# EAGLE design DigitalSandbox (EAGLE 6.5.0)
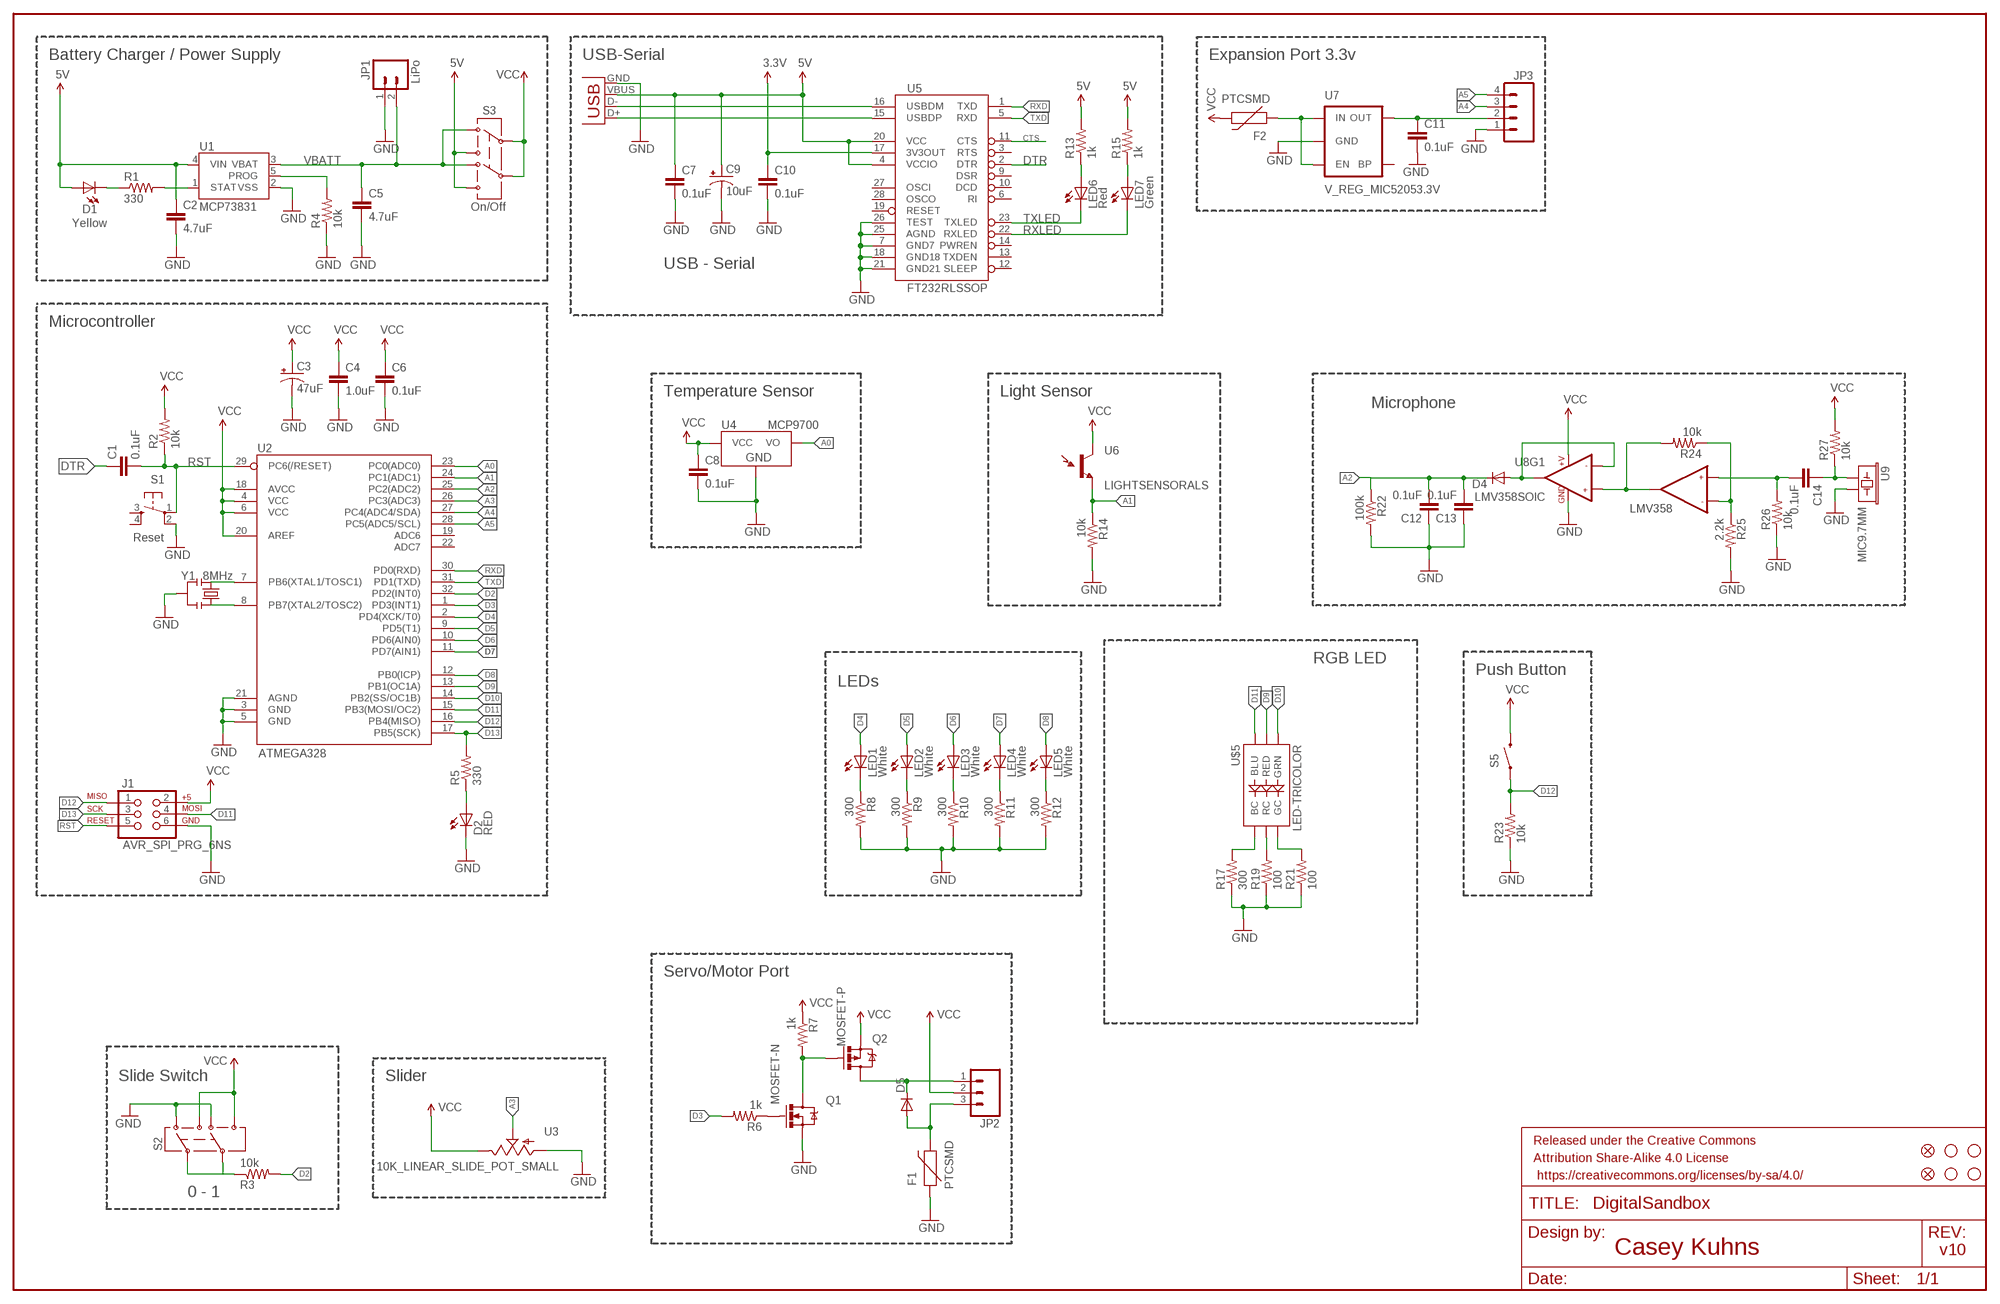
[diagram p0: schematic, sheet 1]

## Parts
C1  0.1uF  0.1UF-25V(+80/-20%)(0603)  [0603-CAP]
C2  4.7uF  4.7UF-6.3V-10%(0603)0603  [0603-CAP]
C3  47uF  47UF-10V-10%(TANT)  [EIA3528]
C4  1.0uF  1.0UF-16V-10%(0603)  [0603-CAP]
C5  4.7uF  4.7UF-6.3V-10%(0603)0603  [0603-CAP]
C6  0.1uF  0.1UF-25V(+80/-20%)(0603)  [0603-CAP]
C7  0.1uF  0.1UF-25V(+80/-20%)(0603)  [0603-CAP]
C8  0.1uF  0.1UF-25V(+80/-20%)(0603)  [0603-CAP]
C9  10uF  10UF-16V-10%(TANT)  [EIA3216]
C10  0.1uF  0.1UF-25V(+80/-20%)(0603)  [0603-CAP]
C11  0.1uF  0.1UF-25V(+80/-20%)(0603)  [0603-CAP]
C12  0.1uF  0.1UF-25V(+80/-20%)(0603)  [0603-CAP]
C13  0.1uF  0.1UF-25V(+80/-20%)(0603)  [0603-CAP]
C14  0.1uF  0.1UF-25V(+80/-20%)(0603)  [0603-CAP]
D1  Yellow  LED-YELLOW0603  [LED-0603]
D2  RED  LED-RED1206  [LED-1206]
D4  DIODESOD  [SOD-323]
D5  DIODESOD  [SOD-323]
F1  PTCSMD  [PTC-1206]
F2  PTCSMD  [PTC-1206]
FID1  FIDUCIAL1X2  [FIDUCIAL-1X2]
FID2  FIDUCIAL1X2  [FIDUCIAL-1X2]
FRAME1  FRAME-LEDGER  [CREATIVE_COMMONS]
J1  AVR_SPI_PRG_6NS  [2X3-NS]
JP1  LiPo  M02-JST-2MM-SMT  [JST-2-SMD]
JP2  M03SMD_RA_FEMALE  [1X03_SMD_RA_FEMALE]
JP3  M04SMD_STRAIGHT_COMBO  [1X04_SMD_STRAIGHT_COMBO]
LED1  White  LED-WHITE  [LED-1206]
LED2  White  LED-WHITE  [LED-1206]
LED3  White  LED-WHITE  [LED-1206]
LED4  White  LED-WHITE  [LED-1206]
LED5  White  LED-WHITE  [LED-1206]
LED6  Red  LED-RED0603  [LED-0603]
LED7  Green  LED-GREEN0603  [LED-0603]
Q1  MOSFET-N  MOSFET-NCHANNELBSS138  [SOT23]
Q2  MOSFET-P  MOSFET-PCHANNEL  [SOT23-3]
R1  330  330OHM1/10W1%(0603)  [0603-RES]
R2  10k  10KOHM1/10W1%(0603)0603  [0603-RES]
R3  10k  10KOHM1/10W1%(0603)0603  [0603-RES]
R4  10k  10KOHM1/10W1%(0603)0603  [0603-RES]
R5  330  330OHM1/10W1%(0603)  [0603-RES]
R6  1k  1KOHM1/10W1%(0603)  [0603-RES]
R7  1k  1KOHM1/10W1%(0603)  [0603-RES]
R8  300  300OHM-1/10W-1%(0603)  [0603-RES]
R9  300  300OHM-1/10W-1%(0603)  [0603-RES]
R10  300  300OHM-1/10W-1%(0603)  [0603-RES]
R11  300  300OHM-1/10W-1%(0603)  [0603-RES]
R12  300  300OHM-1/10W-1%(0603)  [0603-RES]
R13  1k  1KOHM1/10W1%(0603)  [0603-RES]
R14  10k  10KOHM1/10W1%(0603)0603  [0603-RES]
R15  1k  1KOHM1/10W1%(0603)  [0603-RES]
R17  300  300OHM-1/10W-1%(0603)  [0603-RES]
R19  100  100OHM1/10W1%(0603)  [0603-RES]
R21  100  100OHM1/10W1%(0603)  [0603-RES]
R22  100k  100KOHM1/10W1%(0603)  [0603-RES]
R23  10k  10KOHM1/10W1%(0603)0603  [0603-RES]
R24  10k  10KOHM1/10W1%(0603)0603  [0603-RES]
R25  2.2k  2.2KOHM1/10W1%(0603)  [0603-RES]
R26  10k  10KOHM1/10W1%(0603)0603  [0603-RES]
R27  10k  10KOHM1/10W1%(0603)0603  [0603-RES]
S1  Reset  TAC_SWITCHSMD  [TACTILE_SWITCH_SMD]
S2  SWITCH-DPDTAYZ0202  [AYZ0202]
S3  On/Off  SWITCH-DPDTAYZ0202  [AYZ0202]
S5  SWITCH-MOMENTARY-2SMD-4  [TACTILE_SWITCH_TALL]
STANDOFF1  STAND-OFF  [STAND-OFF]
STANDOFF2  STAND-OFF  [STAND-OFF]
STANDOFF3  STAND-OFF  [STAND-OFF]
STANDOFF4  STAND-OFF  [STAND-OFF]
U1  MCP73831  [SOT23-5]
U2  ATMEGA328  ATMEGA328_SMT  [TQFP32-08]
U3  10K_LINEAR_SLIDE_POT_SMALL  [C2031N-1A2-B10K-GP]
U4  MCP9700  MCP9700SMD  [SOT23-3]
U5  FT232RLSSOP  [SSOP28DB]
U6  LIGHTSENSORALS  [ALS-PT19]
U7  V_REG_MIC52053.3V  [SOT23-5]
U8  LMV358SOIC  [SO08]
U9  MIC9.7MM  [MIC-9.7MM]
U$5  LED-TRICOLOR  LED-TRICOLOR-NO-COMPLCC-6-SMD  [PLCC-6-LED]
X1  USBSMD  [USB-MINIB]
Y1  8MHz  RESONATOR8MHZ  [RESONATOR-SMD]

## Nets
3.3V [power]: C10.1 U5.17(3V3OUT)
5V: C2.1 C7.1 C9.A(+) D1.A R13.2 R15.2 S3.3 S3.6 U1.4(VIN) U5.4(VCCIO) U5.20(VCC) X1.VBUS
A0: U2.23(PC0(ADC0)) U4.2(VO)
A1: R14.1 U2.24(PC1(ADC1)) U6.E(E1)
A2: C12.2 C13.2 D4.C R22.1 U2.25(PC2(ADC2))
A3: U2.26(PC3(ADC3)) U3.1(S)
A4: JP3.3 U2.27(PC4(ADC4/SDA))
A5: JP3.4 U2.28(PC5(ADC5/SCL))
BLUE: R17.2 U$5.CB(BC)
CTS: U5.11(CTS)
D2: R3.2 U2.32(PD2(INT0))
D3: R6.2 U2.1(PD3(INT1))
D4: LED1.A U2.2(PD4(XCK/T0))
D5: LED2.A U2.9(PD5(T1))
D6: LED3.A U2.10(PD6(AIN0))
D7: LED4.A U2.11(PD7(AIN1))
D8: LED5.A U2.12(PB0(ICP))
D9: U2.13(PB1(OC1A)) U$5.AR(RED)
D10: U2.14(PB2(SS/OC1B)) U$5.AG(GRN)
D11: J1.4 U2.15(PB3(MOSI/OC2)) U$5.AB(BLU)
D12: J1.1 R23.2 S5.A2 U2.16(PB4(MISO))
D13: J1.3 R5.2 U2.17(PB5(SCK))
DTR: C1.1 U5.2(DTR)
GND [power]: C2.2 C3.C(-) C4.2 C5.2 C6.2 C7.2 C8.2 C9.C(-) C10.2 C11.2 C12.1 C13.1 D2.C F1.1 J1.6 JP1.1 JP3.1 Q1.2(S) R4.1 R8.2 R9.2 R10.2 R11.2 R12.2 R14.2 R17.1 R19.1 R21.1 R22.2 R23.1 R25.2 R26.1 S1.2 S2.1 S2.4 U1.2(VSS) U2.3(GND) U2.5(GND) U2.21(AGND) U3.2(A) U4.3(GND) U5.7(GND7) U5.18(GND18) U5.21(GND21) U5.25(AGND) U5.26(TEST) U7.2(GND) U8.4(GND) U9.2 X1.GND Y1.2
GRN: R21.2 U$5.CG(GC)
N$1: U2.7(PB6(XTAL1/TOSC1)) Y1.1
N$2: D2.A R5.1
N$3: U2.8(PB7(XTAL2/TOSC2)) Y1.3
N$4: Q1.3(D) Q2.1(G) R7.2
N$5: LED6.A R13.1
N$6: LED7.A R15.1
N$7 [power]: F2.1 U7.1(IN) U7.3(EN)
N$8: D5.C JP2.1 Q2.3(D)
N$9: LED3.C R10.1
N$10: Q1.1(G) R6.1
N$11: LED4.C R11.1
N$12: C11.1 JP3.2 U7.5(OUT)
N$13: LED5.C R12.1
N$15: R3.1 S2.2 S2.5
N$16 [power]: D5.A F1.2 JP2.3
N$17: C14.1 R27.1 U9.1
N$18: LED1.C R8.1
N$20: C14.2 R26.2 U8.5(+IN2)
N$21: LED2.C R9.1
N$23: R24.1 R25.1 U8.6(-IN2)
N$24: D4.A U8.1(OUT1) U8.2(-IN1)
N$26: R24.2 U8.3(+IN1) U8.7(OUT2)
N$33: D1.C R1.1
PROG: R4.2 U1.5(PROG)
RED: R19.2 U$5.CR(RC)
RST: C1.2 J1.5 R2.1 S1.1 U2.29(PC6(/RESET))
RXD: U2.30(PD0(RXD)) U5.1(TXD)
RXLED: LED7.C U5.22(RXLED)
STAT: R1.2 U1.1(STAT)
TXD: U2.31(PD1(TXD)) U5.5(RXD)
TXLED: LED6.C U5.23(TXLED)
USB_D+: U5.15(USBDP) X1.D+
USB_D-: U5.16(USBDM) X1.D-
VBATT: C5.1 JP1.2 S3.1 S3.4 U1.3(VBAT)
VCC [power]: C3.A(+) C4.1 C6.1 C8.1 F2.2 J1.2 JP2.2 Q2.2(S) R2.2 R7.1 R27.2 S2.3 S2.6 S3.2 S3.5 S5.B2 U2.4(VCC) U2.6(VCC) U2.18(AVCC) U2.20(AREF) U3.3(E) U4.1(VCC) U6.C(C1) U8.8(+V)
Unconnected: S1.3 S1.4 U2.19(ADC6) U2.22(ADC7) U5.3(RTS) U5.6(RI) U5.9(DSR) U5.10(DCD) U5.12(SLEEP) U5.13(TXDEN) U5.14(PWREN) U5.19(RESET) U5.27(OSCI) U5.28(OSCO) U7.4(BP)

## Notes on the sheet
- Battery Charger / Power Supply | USB-Serial | Expansion Port 3.3v
- USB - Serial
- Microcontroller
- Temperature Sensor | Light Sensor
- Microphone
- LMV358
- RGB LED
- Push Button
- LEDs
- Servo/Motor Port
- Slide Switch | Slider
- 0 - 1
- Casey Kuhns | v10

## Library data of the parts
C1 C6-C8 C10-C14 = SparkFun-Capacitors:0.1UF-25V(+80/-20%)(0603): CAP-00810; PROD_ID: CAP-00810
C2 C5 = SparkFun-Capacitors:4.7UF-6.3V-10%(0603): CAP-08280; PROD_ID: CAP-08280
C3 = SparkFun-Capacitors:47UF-10V-10%(TANT): CAP-08310; PROD_ID: CAP-08310
C4 = SparkFun-Capacitors:1.0UF-16V-10%(0603): CAP-00868; PROD_ID: CAP-00868
C9 = SparkFun-Capacitors:10UF-16V-10%(TANT): CAP-00811; PROD_ID: CAP-00811
D1 = SparkFun-LED:LED-YELLOW: Yellow SMD LEDs; PROD_ID: DIO-09003
D2 = SparkFun-LED:LED-RED: Assorted Red LEDs; PROD_ID: DIO-00809
D4 D5 = SparkFun-DiscreteSemi:DIODE: Diode; PROD_ID: DIO-09646
F1 F2 = SparkFun-PowerIC:PTC: Resettable Fuse PTC; PROD_ID: RES-11150
FID1 FID2 = SparkFun-Aesthetics:FIDUCIAL: Fiducial Alignment Points
FRAME1 = SparkFun-Aesthetics:FRAME-LEDGER: Schematic Frame
J1 = SparkFun-Connectors:AVR_SPI_PRG_6: AVR ISP 6 Pin This is the reduced ISP connector for AVR programming. Common on Arduino. This footprint will take up less PCB space and can be used with a 10-pin to 6-pin adapter such as SKU: BOB-08508
JP1 = SparkFun-Connectors:M02: Standard 2-pin 0.1" header. Use with; PROD_ID: CONN-08352
JP2 = SparkFun-Connectors:M03: Header 3 Standard 3-pin 0.1" header. Use with straight break away headers (SKU : PRT-00116), right angle break away headers (PRT-00553), swiss pins (PRT-00743), machine pins (PRT-00117), and female headers (PRT-00115). Molex polarized connector foot print use with SKU : PRT-08232 with associated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; PROD_ID: CONN-10926; VALUE: 1x3 RA Female .1"
JP3 = SparkFun-Connectors:M04: Header 4 Standard 4-pin 0.1" header. Use with straight break away headers (SKU : PRT-00116), right angle break away headers (PRT-00553), swiss pins (PRT-00743), machine pins (PRT-00117), and female headers (PRT-00115). Molex polarized connector foot print use with SKU : PRT-08231 with associated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
LED1-LED5 = SparkFun-LED:LED-WHITE: White SMD LEDs; PROD_ID: DIO-09955; VALUE: WHITE
LED6 = SparkFun-LED:LED-RED: Assorted Red LEDs; PROD_ID: DIO-00819; VALUE: RED
LED7 = SparkFun-LED:LED-GREEN: Various green LEDs; PROD_ID: DIO-00821; VALUE: GREEN
Q1 = SparkFun-DiscreteSemi:MOSFET-NCHANNEL: Common NMOSFET Parts MFG P/NStore IDProd ID FDD8780TRANS-09984 SI7820DNTRANS-11055 FDS6630AIC-08089 2N7002PWTRANS-11151 FQP30N06L COM-10213TRANS-10060 BSS123LT1GTRANS-08345 BSS138TRANS-00830 BS170 2N7000; PROD_ID: TRANS-00830
Q2 = SparkFun-DiscreteSemi:MOSFET-PCHANNEL: Generic PMOSFET; PROD_ID: TRANS-08285
R1 R5 = SparkFun-Resistors:330OHM1/10W1%(0603): RES-00818; PROD_ID: RES-00818
R2-R4 R14 R23 R24 R26 R27 = SparkFun-Resistors:10KOHM1/10W1%(0603): RES-00824; PROD_ID: RES-00824; VALUE: 10K
R6 R7 R13 R15 = SparkFun-Resistors:1KOHM1/10W1%(0603): RES-07856; PROD_ID: RES-07856; VALUE: 1K
R8-R12 R17 = SparkFun-Resistors:300OHM-1/10W-1%(0603): RES-10328; PROD_ID: RES_10328
R19 R21 = SparkFun-Resistors:100OHM1/10W1%(0603): RES-07863; PROD_ID: RES-07863
R22 = SparkFun-Resistors:100KOHM1/10W1%(0603): RES-07828; PROD_ID: RES-07828
R25 = SparkFun-Resistors:2.2KOHM1/10W1%(0603): RES-08272; PROD_ID: RES-08272
S1 = SparkFun-Electromechanical:TAC_SWITCH: Momentary Switch Button commonly used for reset or general input. Spark Fun Electronics SKU : COM-00097 SMT- SWCH-08247; PROD_ID: SWCH-08247
S2 S3 = SparkFun-Electromechanical:SWITCH-DPDT: DPDT Version of the COM-00597; PROD_ID: SWCH-08179; VALUE: DPDT
S5 = SparkFun-Electromechanical:SWITCH-MOMENTARY-2: Various NO switches- pushbuttons, reed, etc; PROD_ID: SWCH-11966
STANDOFF1-STANDOFF4 = SparkFun-Electromechanical:STAND-OFF: #4 Stand Off
U1 = SparkFun-PowerIC:MCP73831: Miniature single cell, fully integrated Li-Ion, Li-polymer charge management controller http://ww1.microchip.com/downloads/en/DeviceDoc/21984a.pdf IC-09995; PROD_ID: IC-09995
U2 = SparkFun-DigitalIC:ATMEGA328_SMT: 32-Pin Atmega328 part Commonly used on Arduino compatible boards Available in QFP and QFN packages TQFP is IC-09069 QFN is non-stock; PROD_ID: IC-09069; VALUE: ATMEGA328P
U3 = SparkFun-Resistors:10K_LINEAR_SLIDE_POT_SMALL; PROD_ID: RES-11924
U4 = SparkFun-Sensors:MCP9700: Analog-output temperature sensor; PROD_ID: IC-08917
U5 = SparkFun-DigitalIC:FT232RL: USB UART FT232RL 4th Generation USB UART (USB <-> Serial) Controller. Spark Fun Electronics SKU : COM-00650 Production SKU IC-00870; PROD_ID: IC-00870
U6 = SparkFun-Sensors:LIGHTSENSOR: Ambient Light Sensor; PROD_ID: IC-11836
U7 = SparkFun-PowerIC:V_REG_MIC5205: V_REG MIC5219 Standard 3.3V and 5V 150mA LDO voltage regulator in SOT-23 layout. Micrel part MIC5205. BP (by-pass) pin is used to lower output noise with 470pF cap, may be left open.; PROD_ID: VREG-00822; VALUE: 3.3V/150mA
U8 = SparkFun-AnalogIC:LMV358: Jellybean rail-to-rail output op-amp; PROD_ID: IC-09657
U9 = SparkFun-Sensors:MIC: Omni-directional electret microphone. 9.7mm standard diameter.; PROD_ID: COMP-08856
U$5 = SparkFun-LED:LED-TRICOLOR-NO-COM; PROD_ID: DIO-12113
X1 = SparkFun-Connectors:USB: USB Connectors USB-B-PTH is fully proven SKU : PRT-00139/CONN-08278 USB-miniB is fully proven SKU : PRT-00587 USB-A-PCB is untested. USB-A-H is throughly reviewed, but untested. Spark Fun Electronics SKU : PRT-00437 USB-B-SMT is throughly reviewed, but untested. Needs silkscreen touching up.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; PROD_ID: CONN-08193
Y1 = SparkFun-FreqCtrl:RESONATOR: Resonator Small SMD resonator. Used, eg, on the Arduino Pro/ Pro Mini boards. 8MHz- XTAL-08895 16MHz- XTAL-08900; PROD_ID: XTAL-08895; VALUE: 8MHZ

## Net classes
0 default: width 0.203 mm
1 power: width 0.254 mm

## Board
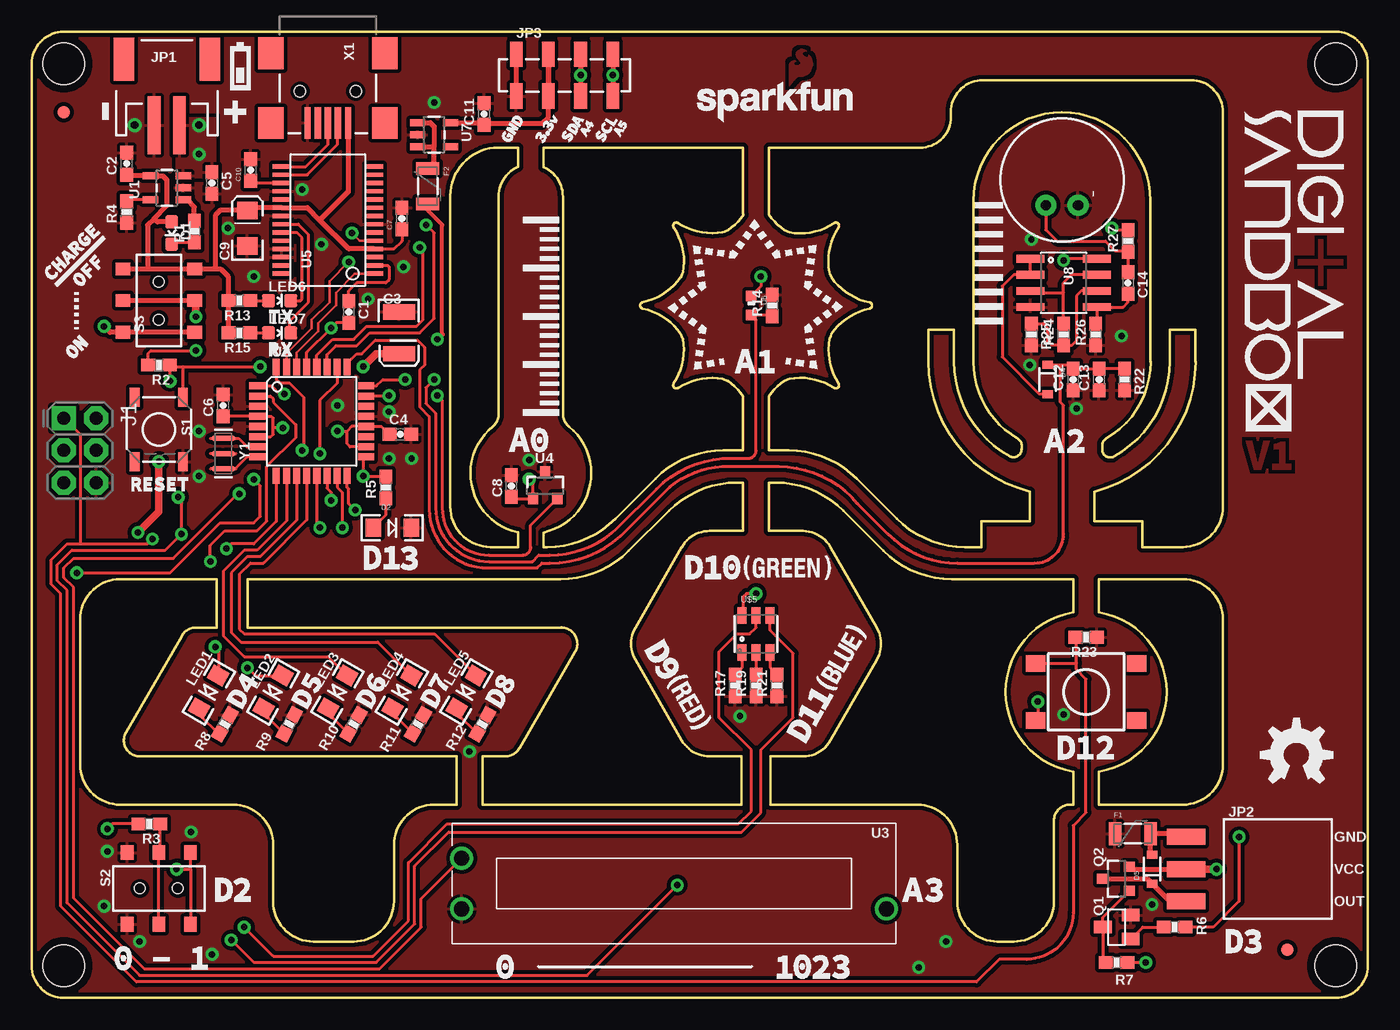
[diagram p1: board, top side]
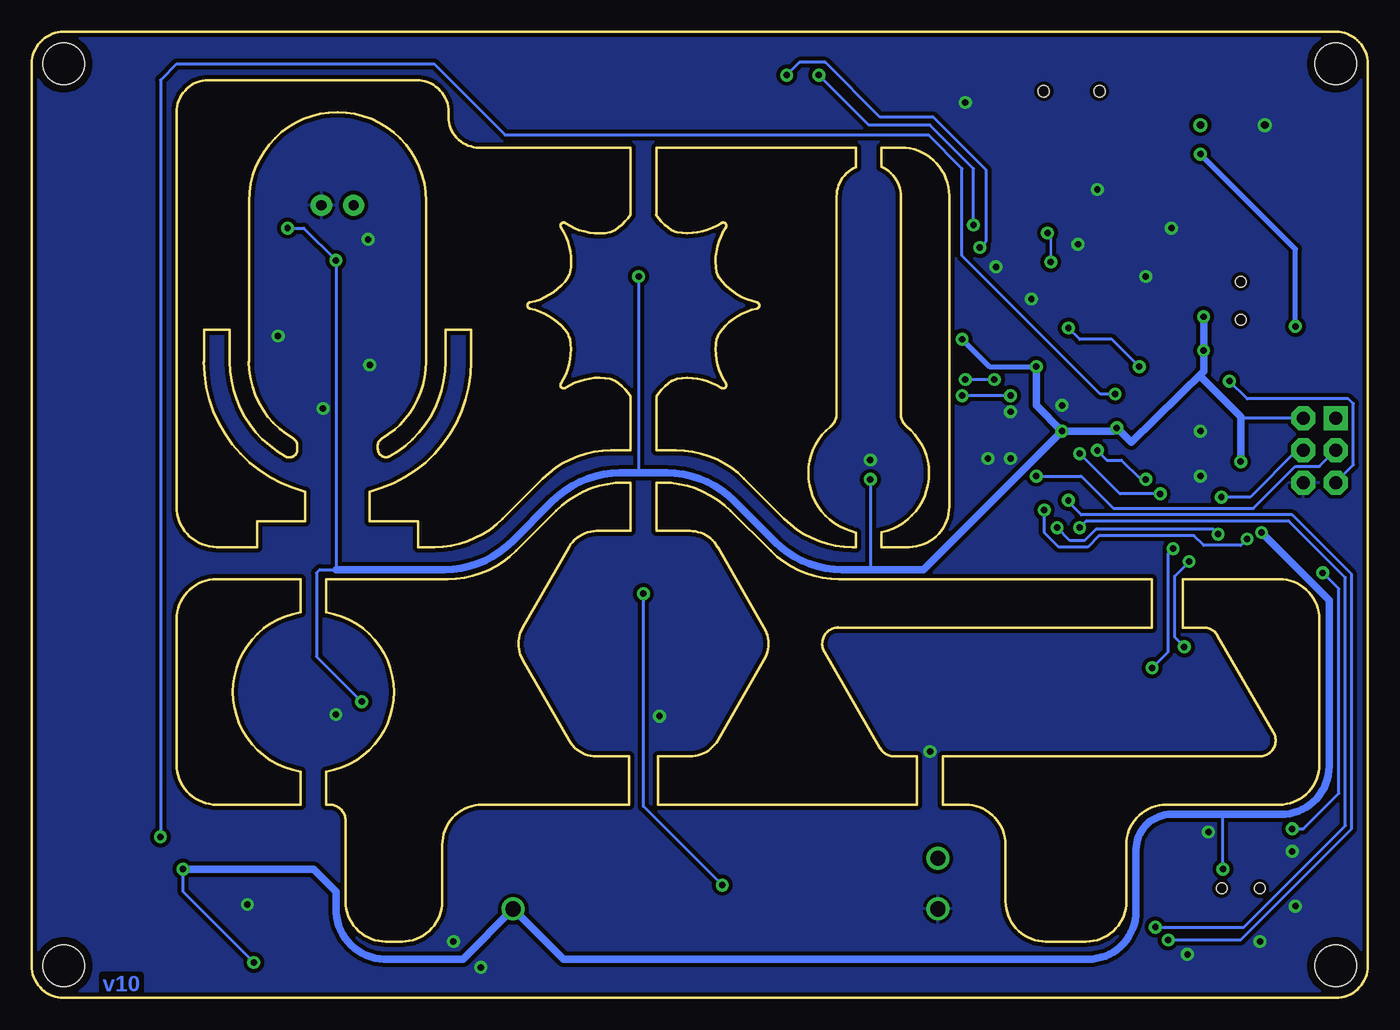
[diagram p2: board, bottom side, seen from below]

Size 105.41 x 76.2 mm. Coordinates in mm from the lower left corner, seen from the top.
Outline: 182 segments
Copper layers (1*16): Top 0.035mm / dielectric 1.5mm / Bottom 0.035mm
Design rules "SparkFun-2-layer": minimum track width 7mil, minimum drill 15mil, track to track 8mil, track to pad 8mil, pad to pad 8mil, via to via 8mil, smd to smd 8mil, copper to edge 8mil, drill to drill 8mil, minimum pad ring 12mil, minimum via ring 10mil, stop-mask expansion 4mil, vias tented up to drill 20mil, thermal gap 10mil

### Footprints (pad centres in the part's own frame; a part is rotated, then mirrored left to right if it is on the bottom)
0603-CAP = smd 1.1 x 1: 1 -0.85,0; 2 0.85,0
EIA3528 = smd 1.2 x 2.5: A 1.65,0; C -1.65,0
EIA3216 = smd 1.4 x 1.6: A 1.4,0; C -1.4,0
LED-0603 = smd 1 x 1: A 0,-0.877; C 0,0.877
LED-1206 = smd 1.2 x 1.4: A -1.5,0; C 1.5,0
SOD-323 = smd 0.63 x 0.83: A 1.15,0; C -1.15,0
PTC-1206 = smd 1 x 1.8: 1 -1.4,0; 2 1.4,0
FIDUCIAL-1X2 = smd 1 x 1: 1 0,0
2X3-NS = drill 1.016 pad 1.88 square: 1 -2.54,-1.27 | drill 1.016 pad 1.88 octagon: 2 -2.54,1.27; 3 0,-1.27; 4 0,1.27; 5 2.54,-1.27; 6 2.54,1.27
JST-2-SMD = smd 1 x 4.6: 1 -1,-3.7; 2 1,-3.7 | smd 1.6 x 3.4: NC1 -3.4,1.5; NC2 3.4,1.5
1X03_SMD_RA_FEMALE = smd 1.25 x 3: 1 -2.54,7.225; 2 0,7.225; 3 2.54,7.225
1X04_SMD_STRAIGHT_COMBO = smd 1 x 2: 1 0,-1.65; 1-2 0,1.65; 2 2.54,1.65; 2-2 2.54,-1.65; 3 5.08,-1.65; 3-2 5.08,1.65; 4 7.62,1.65; 4-2 7.62,-1.65
SOT23 = smd 1 x 1.4: 1 -0.95,-1.1; 2 0.95,-1.1; 3 0,1.1
SOT23-3 = smd 0.8 x 0.9: 1 -0.95,-1; 2 0.95,-1; 3 0,1.1
0603-RES = smd 1.1 x 1: 1 -0.85,0; 2 0.85,0
TACTILE_SWITCH_SMD = smd 1.524 x 0.762: 1 -2.54,1.905; 2 2.54,1.905; 3 -2.54,-1.905; 4 2.54,-1.905
AYZ0202 = smd 1 x 1.15: 1 -2.5,2.825; 2 0,2.825; 3 2.5,2.825; 4 -2.5,-2.825; 5 0,-2.825; 6 2.5,-2.825 | hole 0.85: 1.5,0; -1.5,0
TACTILE_SWITCH_TALL = smd 1.55 x 1.3: A1 -3.975,-2.25; A2 3.975,-2.25; B1 -3.975,2.25; B2 3.975,2.25
STAND-OFF = hole 3.302: 0,0
SOT23-5 = smd 0.55 x 1.2: 1 -0.95,-1.3; 2 0,-1.3; 3 0.95,-1.3; 4 0.95,1.3; 5 -0.95,1.3
TQFP32-08 = smd 1.27 x 0.559: 1 -4.293,2.8; 2 -4.293,2; 3 -4.293,1.2; 4 -4.293,0.4; 5 -4.293,-0.4; 6 -4.293,-1.2; 7 -4.293,-2; 8 -4.293,-2.8; 17 4.293,-2.8; 18 4.293,-2; 19 4.293,-1.2; 20 4.293,-0.4; 21 4.293,0.4; 22 4.293,1.2; 23 4.293,2; 24 4.293,2.8 | smd 0.559 x 1.27: 9 -2.8,-4.293; 10 -2,-4.293; 11 -1.2,-4.293; 12 -0.4,-4.293; 13 0.4,-4.293; 14 1.2,-4.293; 15 2,-4.293; 16 2.8,-4.293; 25 2.8,4.293; 26 2,4.293; 27 1.2,4.293; 28 0.4,4.293; 29 -0.4,4.293; 30 -1.2,4.293; 31 -2,4.293; 32 -2.8,4.293
C2031N-1A2-B10K-GP = drill 1.2: 1 -16.75,2; 2 -16.75,-2; 3 16.75,-2
SSOP28DB = smd 0.348 x 1.397: 1 -4.225,-3.656; 2 -3.575,-3.656; 3 -2.925,-3.656; 4 -2.275,-3.656; 5 -1.625,-3.656; 6 -0.975,-3.656; 7 -0.325,-3.656; 8 0.325,-3.656; 9 0.975,-3.656; 10 1.625,-3.656; 11 2.275,-3.656; 12 2.925,-3.656; 13 3.575,-3.656; 14 4.225,-3.656; 15 4.225,3.656; 16 3.575,3.656; 17 2.925,3.656; 18 2.275,3.656; 19 1.625,3.656; 20 0.975,3.656; 21 0.325,3.656; 22 -0.325,3.656; 23 -0.975,3.656; 24 -1.625,3.656; 25 -2.275,3.656; 26 -2.925,3.656; 27 -3.575,3.656; 28 -4.225,3.656
ALS-PT19 = smd 0.8 x 0.8: C -0.75,0; E 0.75,0
SO08 = smd 0.61 x 2.21: 1 -1.905,-2.616; 2 -0.635,-2.616; 3 0.635,-2.616; 4 1.905,-2.616; 5 1.905,2.616; 6 0.635,2.616; 7 -0.635,2.616; 8 -1.905,2.616
MIC-9.7MM = drill 0.8 pad 1.676: 1 -2,1.27; 2 -2,-1.27
PLCC-6-LED = smd 0.7 x 1.3: AB -1.1,1.475; AG 1.1,1.475; AR 0,1.475; CB -1.1,-1.475; CG 1.1,-1.475; CR 0,-1.475
USB-MINIB = smd 2.5 x 0.5: D+ 2.5,0; D- 2.5,0.8; GND 2.5,-1.6; ID 2.5,-0.8; VBUS 2.5,1.6 | smd 2.5 x 2: MTN1 -3,4.5; MTN2 2.5,4.5; MTN3 -3,-4.5; MTN4 2.5,-4.5 | hole 0.9: 0,2.2; 0,-2.2
RESONATOR-SMD = smd 0.45 x 1.905: 1 -1.2,0; 2 0,0; 3 1.2,0

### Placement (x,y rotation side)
C1  25.02,54.1 270 top
C2  7.49,65.79 90 top
C3  28.99,52.45 270 top
C4  29.08,44.45 0 top
C5  14.22,64.26 270 top
C6  15.11,46.74 90 top
C7  29.21,61.47 90 top
C8  37.85,40.39 90 top
C9  17.02,60.71 90 top
C10  17.27,65.28 90 top
C11  35.69,69.72 90 top
C12  82.17,48.77 90 top
C13  84.2,48.77 90 top
C14  86.49,56.39 270 top
D1  11.05,60.33 180 top
D2  28.45,37.08 0 top
D4  80.14,48.77 270 top
D5  88.39,10.16 90 top
F1  86.87,12.95 0 top
F2  31.24,64.01 270 top
FID1  99.06,3.81 0 top
FID2  2.54,69.85 0 top
FRAME1  not placed on the board
J1  3.81,43.18 270 top
JP1  10.67,72.52 0 top
JP2  98.3,10.16 90 top
JP3  38.23,72.77 0 top
LED1  13.97,24.13 240 top
LED2  19.05,24.13 240 top
LED3  24.13,24.13 240 top
LED4  29.21,24.13 240 top
LED5  34.29,24.13 240 top
LED6  19.56,54.99 270 top
LED7  19.56,52.45 270 top
Q1  85.6,5.59 90 top
Q2  85.6,9.4 90 top
R1  12.83,60.45 90 top
R2  10.03,49.91 180 top
R3  9.27,13.72 180 top
R4  7.49,61.98 90 top
R5  27.94,40.26 90 top
R6  90.17,5.59 0 top
R7  85.6,2.79 180 top
R8  15.24,21.59 60 top
R9  20.32,21.59 62 top
R10  25.4,21.59 60 top
R11  30.48,21.59 60 top
R12  35.56,21.59 60 top
R13  16.38,54.99 180 top
R14  58.42,54.61 90 top
R15  16.38,52.45 180 top
R17  55.5,24.64 90 top
R19  57.15,24.64 90 top
R21  58.8,24.64 90 top
R22  86.23,48.77 270 top
R23  83.19,28.45 180 top
R24  81.41,52.32 90 top
R25  78.87,52.32 270 top
R26  83.95,52.32 90 top
R27  86.49,59.69 90 top
S1  10.03,44.83 270 top
S2  10.03,8.64 0 top
S3  10.03,54.99 90 top
S5  83.19,24.13 180 top
STANDOFF1  102.87,73.66 0 top
STANDOFF2  102.87,2.54 0 top
STANDOFF3  2.54,2.54 0 top
STANDOFF4  2.54,73.66 0 top
U1  10.67,63.88 90 top
U2  22.1,45.47 0 top
U3  50.67,9.02 0 top
U4  40.51,40.39 0 top
U5  23.37,61.34 90 top
U6  56.77,54.61 270 top
U7  31.75,68.07 270 top
U8  81.41,56.39 270 top
U9  81.28,64.52 90 top
U$5  57.15,28.7 0 top
X1  23.37,71.5 270 top
Y1  15.11,42.93 270 top

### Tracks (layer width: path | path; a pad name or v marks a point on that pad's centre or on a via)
3.3V
  Top 0.254: U5.17 17.27,64.27 C10.1 17.27,64.52
5V
  Top 0.254: U5.4 28.59,59.07 29.21,59.69 C7.1
  Top 0.406: C2.1 7.49,64.83 U1.4 10.35,64.83 10.67,64.52 10.67,62.48 9.65,61.47 | D1.A 9.92,61.2 9.65,61.47 | R15.2 R13.2 15.49,55.03 15.49,56.9 14.9,57.49 14.48,57.49 | 14.48,57.49 14.48,61.72 14.86,62.11 C9.A 17.23,62.32 U5.20 21.76,62.32 22.73,61.34 | 9.65,61.47 9.14,60.96 9.14,57.49 | X1.VBUS 24.97,63.58 22.73,61.34 | U5.4 25.01,59.07 22.73,61.34 | 14.48,57.49 S3.6 9.14,57.49 | S3.3 9.14,57.49
A0  (via drill 0.51)
  Top 0.254: U2.23 26.42,47.5 v28.19,47.5 | v32,47.5 32.38,47.12 32.38,38.61 arc90 36.07,34.92 38.73,34.92 arc90 39.37,35.56 39.37,37.29 U4.2
  Bottom 0.254: v28.19,47.5 v32,47.5
A1  (via drill 0.51)
  Top 0.254: R14.1 58.32,53.86 U6.E 57.15,53.48 57.15,43.18 arc-90 56.52,42.55 54.48,42.55 arc40 49.28,40.13 46.23,37.08 arc-44 40.89,34.92 40.01,34.92 39.5,34.42 36.07,34.42 arc-90 31.88,38.61 31.88,46.1 31.11,46.86 31.11,48.13 v31.75,48.77 | U2.24 27.18,48.27 27.69,48.77 v29.46,48.77
  Bottom 0.254: v29.46,48.77 v31.75,48.77
A2
  Top 0.254: R22.1 C13.2 C12.2 arc90 81.87,49.92 81.15,49.92 | U2.25 24.9,50.04 25.65,50.8 26.04,50.8 27.1,51.87 30.43,51.87 30.99,51.31 30.99,49.91 30.61,49.53 30.61,46.61 31.37,45.85 31.37,38.48 arc90 35.94,33.91 39.88,33.91 40.26,34.29 40.89,34.29 arc47 46.99,36.96 49.91,39.88 arc-42 54.48,41.91 58.93,41.91 arc-50 65.15,38.99 67.56,36.58 arc45 73.03,34.29 79.12,34.29 arc90 81.41,36.58 81.41,46.74 81.15,46.99 81.15,49.92 | D4.C 81.15,49.92
A3  (via drill 0.51)
  Top 0.254: U2.26 24.1,48.48 22.73,47.12 v22.73,42.93 | v16.38,39.75 16.26,39.75 11.18,34.67 3.3,34.67 2.54,33.91 2.54,33.15 3.3,32.38 3.3,7.87 8.89,2.29 27.43,2.29 30.73,5.59 30.73,7.83 U3.1
  Bottom 0.254: v22.73,42.93 19.56,39.75 v16.38,39.75 | 34.45,11.02 U3.1
A4  (via drill 0.51)
  Top 0.254: U2.27 23.3,50.73 24,51.44 25.65,51.44 26.67,52.45 30.61,52.45 31.75,53.59 31.75,60.33 v31.11,60.96 | v43.31,72.77 JP3.3
  Bottom 0.254: v31.11,60.96 31.11,65.41 34.54,68.83 39.37,68.83 v43.31,72.77
A5  (via drill 0.51)
  Top 0.254: U2.28 22.5,50.69 23.75,51.94 25.4,51.94 26.42,52.96 30.35,52.96 30.86,53.47 30.86,58.93 v30.61,59.18 | v45.85,72.77 45.85,74.3 45.97,74.42 | JP3.4 45.97,74.42 | 45.97,74.42
  Bottom 0.254: v30.61,59.18 30.1,59.69 30.1,65.28 34.29,69.47 38.48,69.47 42.8,73.79 44.83,73.79 v45.85,72.77
BLUE
  Top 0.254: U$5.CB 56.05,26.04 R17.2
D2  (via drill 0.51)
  Top 0.254: U2.32 19.3,48.77 19.56,48.51 20.32,48.51 21.46,47.37 21.46,43.31 v21.34,43.18 | R3.2 6.35,13.72 v5.97,13.34 | v3.56,33.53 10.92,33.53 14.86,37.47 17.53,37.47 18.03,37.97 18.03,40.39 v17.53,40.89
  Bottom 0.254: v21.34,43.18 20.57,42.42 19.43,42.42 17.91,40.89 v17.53,40.89 | v5.97,13.34 5.08,13.34 2.29,16.13 2.29,32.26 v3.56,33.53
D3  (via drill 0.51)
  Top 0.254: U2.1 18.92,48.26 19.56,47.62 v19.94,47.62 | v95.25,12.7 95.25,7.62 93.22,5.59 R6.2
  Bottom 0.254: v19.94,47.62 21.08,47.62 32,58.55 32,65.41 34.67,68.07 68.07,68.07 73.66,73.66 93.98,73.66 95.25,72.39 v95.25,12.7
D4  (via drill 0.51)
  Top 0.254: U2.2 18.83,47.47 19.05,47.24 19.05,46.99 20.83,45.21 20.83,44.2 18.54,41.91 18.54,37.59 17.78,36.83 15.24,36.83 14.1,35.69 v14.1,34.42 | v14.48,27.69 14.73,27.43 14.73,25.42 | LED1.A 14.73,25.42 | 14.73,25.42 14.73,25.4
  Bottom 0.254: v14.48,27.69 15.24,28.45 15.24,33.27 v14.1,34.42
D5  (via drill 0.51)
  Top 0.254: U2.9 19.3,37.59 17.53,35.81 15.75,35.81 v15.37,35.43 | v17.02,26.04 17.65,25.4 19.81,25.4 19.81,25.42 LED2.A
  Bottom 0.254: v17.02,26.04 15.75,27.3 15.75,35.05 v15.37,35.43
D6
  Top 0.254: U2.10 20.1,37.62 17.78,35.31 16.76,35.31 15.11,33.66 15.11,28.57 16.76,26.92 23.39,26.92 LED3.A
D7
  Top 0.254: U2.11 20.9,37.66 18.03,34.8 17.02,34.8 15.75,33.53 15.75,28.83 16.51,28.07 27.3,28.07 29.96,25.41 | 29.97,25.4 29.96,25.41 | 29.96,25.41 LED4.A
D8
  Top 0.254: U2.12 21.7,37.7 18.29,34.29 17.27,34.29 16.38,33.4 16.38,29.08 16.76,28.7 31.77,28.7 LED5.A
D9  (via drill 0.51)
  Top 0.254: v16.76,5.59 19.05,3.3 26.92,3.3 29.72,6.1 29.72,10.67 32.77,13.72 55.75,13.72 56.77,14.73 56.77,19.56 54.23,22.1 54.23,27.3 55.63,28.7 56.64,28.7 57.15,29.21 U$5.AR | U2.13 22.5,37.32 v22.73,37.08
  Bottom 0.254: v16.76,5.59 9.78,5.59 1.78,13.59 1.78,33.15 6.22,37.59 22.23,37.59 v22.73,37.08
  pour Top: 97.87,42.1 97.87,41.7 99.38,41.7 99.38,42.1 98.9,42.1 98.9,43.82 98.54,43.82 98.51,43.81 98.45,43.77 98.39,43.75 98.36,43.73 98.33,43.72 98.29,43.71 98.26,43.7 98.22,43.68 98.18,43.67 98.15,43.66 98.11,43.65 98.06,43.65 97.98,43.63 97.98,43.32 98.41,43.32 98.41,42.1
D10  (via drill 0.51)
  Top 0.254: v15.75,4.57 17.53,2.79 27.18,2.79 30.23,5.84 30.23,10.41 32.89,13.08 56.01,13.08 57.53,14.61 57.53,19.56 60.07,22.1 60.07,27.18 58.25,29 U$5.AG | U2.14 23.3,40.2 23.62,39.88 v23.62,39.24
  Bottom 0.254: v15.75,4.57 10.03,4.57 1.27,13.34 1.27,33.4 5.97,38.1 22.61,38.1 23.62,39.12 v23.62,39.24 23.62,39.37
D11  (via drill 0.51)
  Top 0.254: U2.15 24.1,40.29 24.51,39.88 v24.51,37.08 | v11.56,39.5 11.81,39.24 v11.81,36.58 10.54,35.31 3.17,35.31 2.03,34.16 2.03,32.89 2.79,32.13 2.79,7.49 8.51,1.78 43.81,1.78 v50.93,8.89 | v57.15,31.88 56.39,31.88 56.13,31.62 56.13,30.22 U$5.AB
  Bottom 0.254: v11.81,36.58 12.19,36.96 21.46,36.96 22.35,36.07 23.5,36.07 v24.51,37.08 | J1.4 5.59,43.18 9.27,39.5 v11.56,39.5 | v50.93,8.89 57.15,15.11 v57.15,31.88
D12  (via drill 0.51)
  Top 0.254: 3.81,35.81 2.79,35.81 1.52,34.54 1.52,32.64 2.29,31.88 2.29,7.24 8.26,1.27 74.55,1.27 76.33,3.05 78.49,3.05 arc90 82.17,6.73 82.17,13.59 83.19,14.61 83.19,25.15 82.42,25.91 82.42,26.42 | 3.81,35.81 9.14,35.81 v9.53,36.2 | v25.53,38.48 25.02,38.99 25.02,40.13 24.9,40.25 U2.16 | J1.1 3.81,44.45 3.81,35.81 | 82.42,26.42 82.42,28.36 R23.2 | S5.A2 82.39,26.38 82.42,26.42
  Bottom 0.254: v9.53,36.2 10.03,35.69 12.95,35.69 13.72,36.45 21.21,36.45 22.1,35.56 24.38,35.56 25.53,36.7 v25.53,38.48
D13  (via drill 0.51)
  Top 0.254: U2.17 26.16,42.44 v26.16,41.15 27.94,41.15 R5.2
  Bottom 0.254: v26.16,41.15 22.61,41.15 20.07,38.61 9.02,38.61 5.71,41.91 3.81,41.91 J1.3
DTR
  Top 0.254: U5.2 28.09,57.77 28.19,57.66 28.19,56.64 27.94,56.39 25.65,56.39 25.02,55.75 C1.1
GND  (via drill 0.51, 0.6)
  other vias: 21.34,63.75 22.86,59.44 15.49,60.71 17.53,56.9 13.21,44.7 34.54,19.43 82.42,46.48 78.74,49.91 85.98,52.2 78.87,59.82 29.97,42.55 28.19,42.55 14.22,3.43 72.14,4.45 69.98,2.41 39.24,42.42 29.34,57.66 26.54,55.12 31.75,70.61 13.21,41.15 28.19,46.23 24.13,46.74 81.41,22.35 8.51,4.45 5.71,7.24 5.97,11.56 12.57,13.08 8.13,68.83 88.39,7.37 55.88,22.23
  pour Top (isolate 0.305, rank 6): 105.41,76.2 0,76.2 0,0 105.41,0
  pour Bottom (isolate 0.305, rank 6): 105.41,76.2 0,76.2 0,0 105.41,0
GRN
  Top 0.254: U$5.CG 58.25,26.04 R21.2
N$1
  Top 0.254: Y1.1 16.33,44.13 16.99,43.47 U2.7
N$2
  Top 0.254: R5.1 27.94,38.08 D2.A
N$3
  Top 0.254: U2.8 17.01,42.67 16.07,41.73 Y1.3
N$4
  Top 0.254: Q2.1 84.5,6.35 Q1.3 84.5,3.04 R7.2
N$5
  Top 0.254: R13.1 LED6.A
N$6
  Top 0.254: R15.1 LED7.A
N$7
  Top 0.406: U7.1 31.43,69.02 31.75,68.71 31.75,67.18 31.69,67.12 | U7.3 31.69,67.12 | 31.69,67.12 31.69,65.86 F2.1
N$8
  Top 0.406: Q2.3 88,9.4 D5.C 89.78,7.62 JP2.1
N$9
  Top 0.254: LED3.C 23.38,22.45 R10.1
N$10
  Top 0.254: Q1.1 87.65,5.59 R6.1
N$11
  Top 0.254: LED4.C 28.46,22.45 R11.1
N$12
  Top 0.406: JP3.2 40.77,69.47 40.26,68.96 35.94,68.96 35.85,68.87 C11.1 35.54,69.02 U7.5
N$13
  Top 0.254: LED5.C 33.54,22.45 R12.1
N$14
  pour Top: 101.89,57.81 103.49,57.81 103.49,58.21 101.89,58.21 101.89,59.8 101.49,59.8 101.49,58.21 99.89,58.21 99.89,57.81 101.49,57.81 101.49,56.21 101.89,56.21
N$15
  Top 0.254: 10.12,5.72 10.03,5.72 S2.5 S2.2 10.12,11.46 R3.1
N$16
  Top 0.406: JP2.3 90.82,12.95 F1.2 88.27,11.43 D5.A
N$17
  Top 0.254: U9.1 80.01,60.58 80.9,59.69 84.71,59.69 85.47,58.93 86.4,58.93 R27.1 C14.1
N$18
  Top 0.254: LED1.C 13.22,22.34 14.73,20.83 14.79,20.83 R8.1
N$19
  pour Top: 61.26,74.36 61.27,74.25 61.26,74.24 61.26,74.22 61.25,74.21 61.24,74.19 61.18,74.16 61.12,74.16 61.1,74.17 61.08,74.17 61,74.21 60.98,74.23 60.96,74.24 60.94,74.26 60.92,74.27 60.9,74.29 60.88,74.3 60.87,74.32 60.85,74.34 60.82,74.4 60.81,74.41 60.8,74.43 60.8,74.5 60.81,74.52 60.81,74.53 60.82,74.55 60.83,74.56 60.84,74.58 60.89,74.63 60.92,74.64 60.96,74.66 60.99,74.67 61.01,74.67 61.03,74.68 61.09,74.68 61.11,74.67 61.13,74.67 61.12,74.68 61.1,74.69 61.08,74.71 61.05,74.73 61.01,74.75 60.97,74.76 60.93,74.78 60.88,74.79 60.82,74.8 60.77,74.81 60.71,74.81 60.65,74.8 60.59,74.78 60.52,74.75 60.46,74.71 60.41,74.67 60.37,74.62 60.33,74.58 60.31,74.53 60.29,74.49 60.27,74.39 60.29,74.29 60.31,74.25 60.33,74.2 60.36,74.15 60.44,74.05 60.49,74.01 60.58,73.92 60.61,73.88 60.63,73.83 60.65,73.79 60.65,73.68 60.63,73.64 60.61,73.61 60.58,73.58 60.52,73.54 60.48,73.52 60.44,73.51 60.34,73.51 60.31,73.52 60.28,73.52 60.26,73.53 60.23,73.54 60.21,73.56 60.19,73.57 60.18,73.59 60.15,73.62 60.13,73.66 60.13,73.73 60.14,73.75 60.15,73.76 60.15,73.78 60.16,73.79 60.18,73.8 60.2,73.82 60.22,73.83 60.24,73.85 60.25,73.85 60.27,73.86 60.28,73.87 60.29,73.87 60.28,73.88 60.26,73.88 60.24,73.89 60.08,73.89 59.96,73.85 59.93,73.83 59.91,73.82 59.88,73.8 59.84,73.76 59.82,73.73 59.8,73.71 59.78,73.67 59.77,73.64 59.75,73.6 59.74,73.56 59.74,73.52 59.73,73.47 59.73,73.36 59.76,71.92 59.77,71.92 59.77,71.93 59.79,71.95 59.8,71.97 59.82,71.99 59.84,72.02 59.89,72.07 59.91,72.1 59.94,72.14 60,72.2 60.09,72.32 60.13,72.36 60.16,72.4 60.2,72.43 60.23,72.47 60.26,72.5 60.28,72.53 60.31,72.56 60.34,72.58 60.37,72.61 60.4,72.63 60.42,72.64 60.45,72.66 60.49,72.67 60.52,72.67 60.56,72.68 60.74,72.68 60.8,72.69 60.87,72.7 61.05,72.76 61.11,72.79 61.16,72.82 61.26,72.9 61.3,72.94 61.35,72.98 61.43,73.08 61.46,73.13 61.52,73.24 61.57,73.34 61.6,73.44 61.62,73.55 61.63,73.65 61.63,73.74 61.61,73.84 61.59,73.92 61.57,74.01 61.53,74.08 61.5,74.15 61.45,74.21 61.41,74.27 61.36,74.31 61.31,74.34
N$20
  Top 0.254: R26.2 84.02,53.25 U8.5 86.11,54.48 86.49,54.86 C14.2
N$21
  Top 0.254: LED2.C 18.3,22.46 R9.1
N$22
  pour Top: 97.67,43.88 97.17,43.88 96.92,42.86 96.91,42.82 96.89,42.78 96.88,42.73 96.86,42.65 96.85,42.6 96.83,42.52 96.82,42.47 96.8,42.39 96.79,42.34 96.78,42.3 96.76,42.26 96.75,42.21 96.74,42.17 96.73,42.17 96.72,42.21 96.7,42.26 96.68,42.34 96.67,42.39 96.65,42.47 96.64,42.52 96.62,42.6 96.61,42.65 96.59,42.73 96.58,42.78 96.57,42.82 96.55,42.86 96.29,43.88 95.77,43.88 96.43,41.7 97.02,41.7
N$23
  Top 0.254: U8.6 82.8,55.75 82.42,55.37 82.42,51.82 82.08,51.47 R24.1 80.48,51.47 80.14,51.82 80.14,52.83 79.8,53.17 R25.1
N$24
  Top 0.254: U8.1 U8.2 77.47,57.02 76.58,56.13 76.58,50.55 79.51,47.62 D4.A
N$26
  Top 0.254: R24.2 81.41,55.63 | 81.41,55.63 81.41,56.39 82.04,57.02 U8.7 | U8.3 78.79,55.63 81.41,55.63
N$33
  Top 0.254: D1.C 11.08,59.6 R1.1
PROG
  Top 0.254: U1.5 7.6,62.93 R4.2
RED
  Top 0.254: U$5.CR R19.2
RST  (via drill 0.51)
  Top 0.254: U2.29 21.7,50.91 v23.62,52.83 24.04,53.25 C1.2 | S1.1 11.94,49.78 | 11.94,49.78 11.01,49.78 R2.1 10.92,49.87 v10.92,48.64 | 11.94,49.78 v18.03,49.78
  Bottom 0.254: v18.03,49.78 20.19,51.94 22.73,51.94 v23.62,52.83 | J1.5 1.14,42.04 1.14,46.86 1.52,47.24 9.53,47.24 v10.92,48.64
RXD
  Top 0.203: U5.1 25.49,57.12 24,55.63 24,54.61 22.61,53.21 22.61,52.58 20.9,50.87 U2.30
RXLED
  Top 0.254: LED7.C 20.31,53.33 21.84,54.86 21.84,60.2 21.03,61.02 U5.22
STAT
  Top 0.406: U1.1 12.25,62.93 12.83,62.36 R1.2
TXD  (via drill 0.51)
  Top 0.203: U2.31 20.1,50.83 22.1,52.83 22.1,53.47 23.5,54.86 23.5,56.52 v25.02,58.04 | v25.27,60.33 25.88,59.72 U5.5
  Bottom 0.203: v25.02,58.04 25.02,60.07 v25.27,60.33
TXLED
  Top 0.254: LED6.C 21.21,54.99 21.34,55.12 21.34,59.94 20.91,60.37 U5.23
USB_D+
  Top 0.254: U5.15 21.62,65.57 23.37,67.31 X1.D+
USB_D-
  Top 0.254: U5.16 21.74,64.92 24.13,67.31 24.13,68.96 X1.D-
VBATT  (via drill 0.51, 0.6)
  Top 0.406: S3.1 S3.4 6.18,52.49 v5.71,52.96
  Bottom 0.406: v5.71,52.96 5.71,59.05 v13.21,66.55
  other vias: 13.21,68.83
  pour Top (isolate 0.305, rank 2): 11.43,64.77 14.48,64.77 14.48,69.34 11.43,69.34
VCC  (via drill 0.51)
  Top 0.254: C6.1 15.13,45.87 U2.4 18.9,45.87 19.05,45.72 19.05,44.96 | U2.6 18.87,44.27 19.05,44.45 19.05,44.96 | 24.89,44.7 25.25,45.07 U2.20 27.58,45.07 28.19,44.45 C4.1 | U2.18 25.11,43.47 24.89,43.69 24.89,44.7 | v24.13,44.7 24.89,44.7 | v19.81,44.96 19.05,44.96 | v39.24,40.89 39.56,40.57 U4.1 38,39.39 C8.1 | R27.2 85.38,60.54 v85.22,60.71 | U8.8 81.53,58.29 v81.41,58.17 | v11.43,10.16 12.53,10.16 | v93.47,10.16 93.18,9.87 | C3.A 28.96,50.8 | v57.53,56.9 57.53,56.12 U6.C | R2.2 9.18,50.84 9.4,51.05 v12.95,51.05 | R7.1 v87.88,2.79 | v79.38,23.37 79.38,22.05 S5.B2 | 12.53,10.16 S2.3 | 12.53,10.16 S2.6
  Top 0.305: 32.38,52.32 32.38,60.96 31.24,62.1 F2.2
  Top 0.406: S3.5 S3.2 | 32.38,52.32 v32,51.94 | Q2.2 86.79,10.16 JP2.2
  Top 0.61: v12.95,53.72 12.95,54.86 12.88,54.94 arc-45 S3.5 | v26.16,49.78 27.18,50.8 28.96,50.8 | v93.47,10.16 JP2.2 | v10.03,42.29 10.03,38.35 v8.38,36.7
  Bottom 0.254: v39.24,40.89 39.24,33.78 | v57.53,56.9 57.53,41.4 | v85.22,60.71 83.95,60.71 v81.41,58.17 81.41,33.78 82.68,33.78 82.93,33.53 82.93,26.92 v79.38,23.37 | v11.43,10.16 11.43,14.48 11.18,14.48 | J1.2 9.91,45.72 10.03,45.85 | v87.88,2.79 93.47,8.38 v93.47,10.16 | 57.15,41.4 56.9,41.4
  Bottom 0.406: v32,51.94 29.84,49.78 v26.16,49.78
  Bottom 0.61: v24.13,44.7 20.07,44.7 v19.81,44.96 18.67,43.81 12.95,49.4 | 81.41,33.78 72.83,33.78 arc-45 67.53,35.98 64.3,39.2 arc45 59,41.4 57.53,41.4 56.9,41.4 55.3,41.4 arc45 50,39.2 46.77,35.98 arc-45 41.47,33.78 39.24,33.78 35.05,33.78 v24.13,44.7 | v93.47,10.16 83.19,10.16 81.41,8.38 81.41,7.11 arc-90 77.6,3.05 71.39,3.05 U3.3 63.45,3.05 22.1,3.05 arc-90 18.29,6.86 18.29,11.68 arc90 15.49,14.48 11.18,14.48 6.86,14.48 arc-90 3.05,18.29 3.05,31.37 v8.38,36.7 | v26.16,49.78 26.16,46.74 v24.13,44.7 | v12.95,53.72 v12.95,51.05 12.95,49.4 | 12.95,49.4 13.21,49.15 13.21,49.02 10.03,45.85 v10.03,42.29

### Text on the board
Bottom: v10
tPlace: GND | VCC | OUT
tNames: Casey Kuhns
